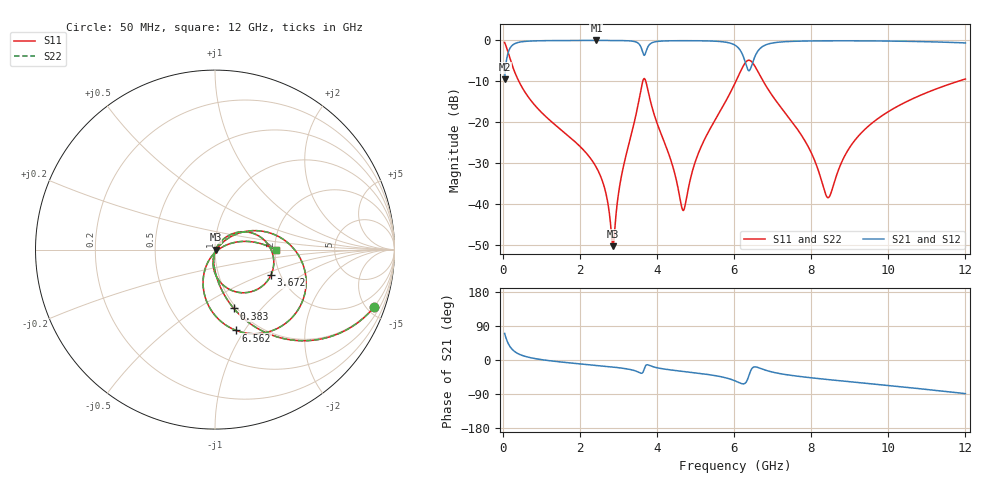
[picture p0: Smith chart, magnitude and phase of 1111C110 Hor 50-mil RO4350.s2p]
# GHz S MA R 50
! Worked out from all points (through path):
!   11951 points, 50 MHz to 12 GHz, reference 50 ohm
!   highest |S21| = -0.02 dB at 2.43 GHz (marker M1); lowest = -9.5 dB at 50 MHz (marker M2)
!   group delay of S21, straight-line fit = 21.6 ps
!   lowest |S11| = -50.2 dB at 2.86 GHz (marker M3), VSWR 1.01, Z = 50.3 - j0.122 ohm
!   |S11| at or under -10 dB: 420.4 MHz to 3.631 GHz (3.211 GHz wide, 158 % of centre); 3.712 GHz to 6.047 GHz (2.335 GHz wide, 47.9 % of centre); 6.759 GHz to 11.8 GHz (5.042 GHz wide, 54.3 % of centre)
!   |S22| runs from -50.2 to -0.5 dB; largest |S21 - S12| = 0
!   S11 on the Smith chart (normalised r, x): 50 MHz: 0.97, -5.56; 383 MHz: 0.97, -0.72; 3.672 GHz: 1.78, -0.58; 6.562 GHz: 0.80, -0.92; 12 GHz: 2.02, -0.01
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0.05  0.9427 -19.8  0.3337 70.2  0.3337 70.2  0.9427 -19.8
0.211  0.5555 -57.6  0.8311 32.3  0.8311 32.3  0.5555 -57.6
0.383  0.344 -72.3  0.9384 17.6  0.9384 17.6  0.344 -72.3
2.042  0.04898 -99.0  0.9973 -10.6  0.9973 -10.6  0.04898 -99.0
2.43  0.02826 -100.7  0.9977 -14.3  0.9977 -14.3  0.02826 -100.7
2.666  0.01437 -97.5  0.9974 -16.6  0.9974 -16.6  0.01437 -97.5
2.86  0.003101 -23.0  0.9967 -18.7  0.9967 -18.7  0.003101 -23.0
3.097  0.02437 55.3  0.994 -21.6  0.994 -21.6  0.02437 55.3
3.54  0.1932 30.9  0.8996 -33.0  0.8996 -33.0  0.1932 30.9
3.672  0.3428 -24.7  0.6571 -23.4  0.6571 -23.4  0.3428 -24.7
4.034  0.08941 -96.4  0.9733 -21.2  0.9733 -21.2  0.08941 -96.4
4.689  0.008464 -24.6  0.9913 -30.2  0.9913 -30.2  0.008464 -24.6
5.103  0.04527 42.5  0.9891 -35.2  0.9891 -35.2  0.04527 42.5
6.025  0.3007 19.2  0.8747 -55.0  0.8747 -55.0  0.3007 19.2
6.314  0.5492 -23.0  0.4998 -58.4  0.4998 -58.4  0.5492 -23.0
6.562  0.4656 -75.3  0.667 -18.2  0.667 -18.2  0.4656 -75.3
6.896  0.248 -104.2  0.906 -29.3  0.906 -29.3  0.248 -104.2
8.017  0.0413 -116.4  0.9842 -47.1  0.9842 -47.1  0.0413 -116.4
8.452  0.01215 -43.3  0.9876 -51.8  0.9876 -51.8  0.01215 -43.3
9.051  0.05378 21.1  0.9878 -57.8  0.9878 -57.8  0.05378 21.1
10.009  0.136 18.6  0.9809 -67.4  0.9809 -67.4  0.136 18.6
12  0.3384 -0.4  0.9309 -88.7  0.9309 -88.7  0.3384 -0.4
